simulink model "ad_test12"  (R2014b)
settings: Solver=ode45  StartTime=0.0  StopTime=10  MaxStep=1e-4  RelTol=1e-3
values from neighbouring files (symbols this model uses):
  ampl = 1    [abtast_rate_1.m]    (also in ad_test_12.m; ad_test_2.m; ad_test_3.m; fft_1.m = 10)
  fsig = 100    [abtast_rate_1.m]    (also in ad_test_12.m = ',num2str(fsig),'; ad_test_2.m = ',num2str(fsig),'; ad_test_3.m = ',num2str(fsig),'; leakage_2.m = 100.5)
  N = 4*1024    (= 4096)    [ad_test_12.m]    (also in ad_test_2.m; ad_test_3.m; DA_wandler_spektr_1.m = 1000; DA_wandler_spektr_2.m = 1024)
  Ts = 1/fs    (= 0.00025)    [abtast_rate_1.m]    (also in ad_test_12.m = 0.0009765625; ad_test_2.m = 0.00048828125; ad_test_3.m = 0.00048828125; DA_wandler_spektr_1.m = 0.01)
undefined symbols (not defined in the file or in its folder): get
libraries: dspspect3 x1, dspstat3 x1, dspsnks4 x1

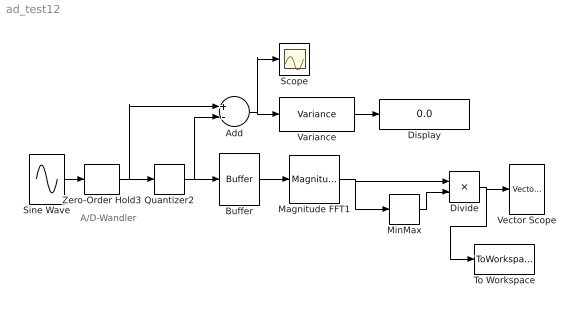
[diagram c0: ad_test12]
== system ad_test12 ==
  note: A/D-Wandler
  Add : Sum  Inputs=+-
  Buffer : Buffer  N=N  ic=eps*ones(N,1)  TreatMby1Signals=One channel
  Display : Display
  Divide : Product  Inputs=*/
  Magnitude FFT1 : dspspect3/Magnitude FFT  mag_or_magsq=Magnitude squared  FFTImplementation=FFTW  fftLenInherit=off  fftsize=N  WrapInput=on
  MinMax : MinMax  Function=max  OutDataTypeStr=double
  Quantizer2 : Quantizer  QuantizationInterval=q  LinearizeAsGain=off  SampleTime=Ts
  Scope : Scope
  Sine Wave : Sin  Amplitude=ampl  Frequency=2*pi*fsig  SampleTime=0
  To Workspace : ToWorkspace  VariableName=Y  SampleTime=-1
  Variance : dspstat3/Variance  run=on  reset_popup=None  InputProcessing=Columns as channels (frame based)  directionMode=Each column  dimension=1  treatSBRowAsCol=on  roiEnable=off  roiType=Rectangles  roiPortion=Entire ROI  roiOutput=Individual statistics for each ROI  roiFlag=off  roundingMode=Floor  overflowMode=off
  Vector Scope : dspsnks4/Vector Scope  ScopeProperties=on  Domain=Frequency  HorizSpan=1  DisplayProperties=off  AxisGrid=on  Memory=off  FrameNumber=on  AxisLegend=off  AxisZoom=off  OpenScopeAtSimStart=on  OpenScopeImmediately=off  FigPos=get(0,'defaultfigureposition')  AxisProperties=off  XUnits=Hertz  XRange=[0...Fs]  InheritXIncr=off  XIncr=Ts  XLabel=Time  XLimit=Auto  XMin=4.2733  XMax=1026.1311  XStart=0  YUnits=dB  YLabel=Leistung in dB  LineProperties=off  XAxisParamsVer=6.9
  Zero-Order Hold3 : ZeroOrderHold  SampleTime=Ts
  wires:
  Buffer/1 -> Magnitude FFT1/1
  Sine Wave/1 -> Zero-Order Hold3/1
  Variance/1 -> Display/1
  Magnitude FFT1/1 -> MinMax/1, Divide/1
  Divide/1 -> To Workspace/1, Vector Scope/1
  MinMax/1 -> Divide/2
  Add/1 -> Scope/1, Variance/1
  Zero-Order Hold3/1 -> Quantizer2/1, Add/1
  Quantizer2/1 -> Add/2, Buffer/1
